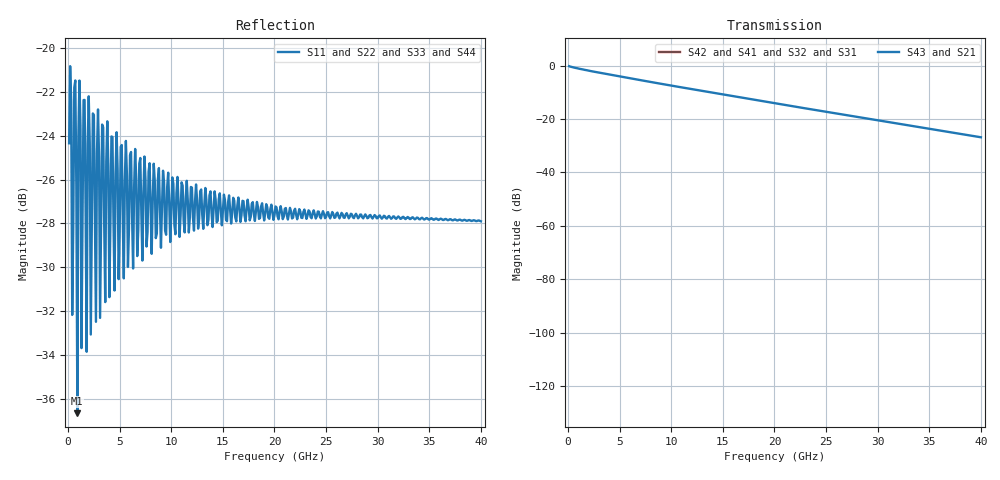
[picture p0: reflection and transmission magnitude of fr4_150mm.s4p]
! Touchstone Ver. 1.0
! Number of ports is 4
! port1 ->  port2
! port3 ->  port4
# Hz	S	RI	R	50.000000
! SCATTERING PARAMETERS  :
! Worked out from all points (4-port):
!   400 points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, 100 MHz to 40 GHz, reference 50 ohm
!   strongest paths, dB at 100 MHz, 10.1 GHz, 20.1 GHz, 30.1 GHz, 40 GHz:
!     S43: -0.2, -7.6, -14.2, -20.5, -26.9
!     S21: -0.2, -7.6, -14.2, -20.5, -26.9
!     S42: -, -, -, -, -
!     S41: -, -, -, -, -
!     S32: -, -, -, -, -
!     S31: -, -, -, -, -
!   lowest |S11| = -36.7 dB at 900 MHz (marker M1), VSWR 1.03, Z = 48.9 - j0.918 ohm
!   |S11| at or under -10 dB: start of sweep to end of sweep
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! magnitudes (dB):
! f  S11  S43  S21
! 100 MHz  -24.3  -0.2  -0.2
! 700 MHz  -21.5  -0.9  -0.9
! 900 MHz  -36.7  -1.0  -1.0
! 1.1 GHz  -21.5  -1.2  -1.2
! 1.8 GHz  -33.9  -1.7  -1.7
! 2 GHz  -22.2  -1.9  -1.9
! 40 GHz  -27.9  -26.9  -26.9
